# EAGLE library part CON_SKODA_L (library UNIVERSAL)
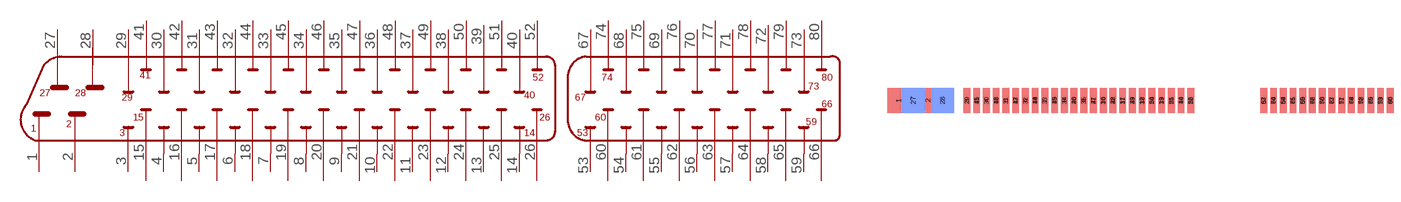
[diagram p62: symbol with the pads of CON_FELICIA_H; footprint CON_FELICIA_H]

Designator prefix CON

## CON_SKODA_L  [CON_FELICIA_H]
1  P$1
2  P$2
3  P$3
4  P$4
5  P$5
6  P$6
7  P$7
8  P$8
9  P$9
10  P$10
11  P$11
12  P$12
13  P$13
14  P$14
15  P$15
16  P$16
17  P$17
18  P$18
19  P$19
20  P$20
21  P$21
22  P$22
23  P$23
24  P$24
25  P$25
26  P$26
27  P$27
28  P$28
29  P$29
30  P$30
31  P$31
32  P$32
33  P$33
34  P$34
35  P$35
36  P$36
37  P$37
38  P$38
39  P$39
40  P$40
41  P$41
42  P$42
43  P$43
44  P$44
45  P$45
46  P$46
47  P$47
48  P$48
49  P$49
50  P$50
51  P$51
52  P$52
53  P$53
54  P$54
55  P$55
56  P$56
57  P$57
58  P$58
59  P$59
60  P$60
61  P$61
62  P$62
63  P$63
64  P$64
65  P$65
66  P$66
67  P$67
68  P$68
69  P$69
70  P$70
71  P$71
72  P$72
73  P$73
74  P$74
75  P$75
76  P$76
77  P$77
78  P$78
79  P$79
80  P$80

## Footprint CON_FELICIA_H (pad centres in mm)
smd 5 x 5.5: 1 -14.98,0.535; 2 -8.56,0.535
smd 1.5 x 5.5 bottom: 3 0,0.535; 4 4.28,0.535; 5 8.56,0.535; 6 12.84,0.535; 7 17.12,0.535; 8 21.4,0.535; 9 25.68,0.535; 10 29.96,0.535; 11 34.24,0.535; 12 38.52,0.535; 13 42.8,0.535; 14 47.08,0.535; 15 2.14,0.535; 16 6.42,0.535; 17 10.7,0.535; 18 14.98,0.535; 19 19.26,0.535; 20 23.54,0.535; 21 27.82,0.535; 22 32.1,0.535; 23 36.38,0.535; 24 40.66,0.535; 25 44.94,0.535; 26 49.22,0.535; 53 65.27,0.535; 54 69.55,0.535; 55 73.83,0.535; 56 78.11,0.535; 57 82.39,0.535; 58 86.67,0.535; 59 90.95,0.535; 60 67.41,0.535; 61 71.69,0.535; 62 75.97,0.535; 63 80.25,0.535; 64 84.53,0.535; 65 88.81,0.535; 66 93.09,0.535
smd 5 x 5.5 bottom: 27 -11.77,0.535; 28 -5.35,0.535
smd 1.5 x 5.5: 29 0,0.535; 30 4.28,0.535; 31 8.56,0.535; 32 12.84,0.535; 33 17.12,0.535; 34 21.4,0.535; 35 25.68,0.535; 36 29.96,0.535; 37 34.24,0.535; 38 38.52,0.535; 39 42.8,0.535; 40 47.08,0.535; 41 2.14,0.535; 42 6.42,0.535; 43 10.7,0.535; 44 14.98,0.535; 45 19.26,0.535; 46 23.54,0.535; 47 27.82,0.535; 48 32.1,0.535; 49 36.38,0.535; 50 40.66,0.535; 51 44.94,0.535; 52 49.22,0.535; 67 65.27,0.535; 68 69.55,0.535; 69 73.83,0.535; 70 78.11,0.535; 71 82.39,0.535; 72 86.67,0.535; 73 90.95,0.535; 74 67.41,0.535; 75 71.69,0.535; 76 75.97,0.535; 77 80.25,0.535; 78 84.53,0.535; 79 88.81,0.535; 80 93.09,0.535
